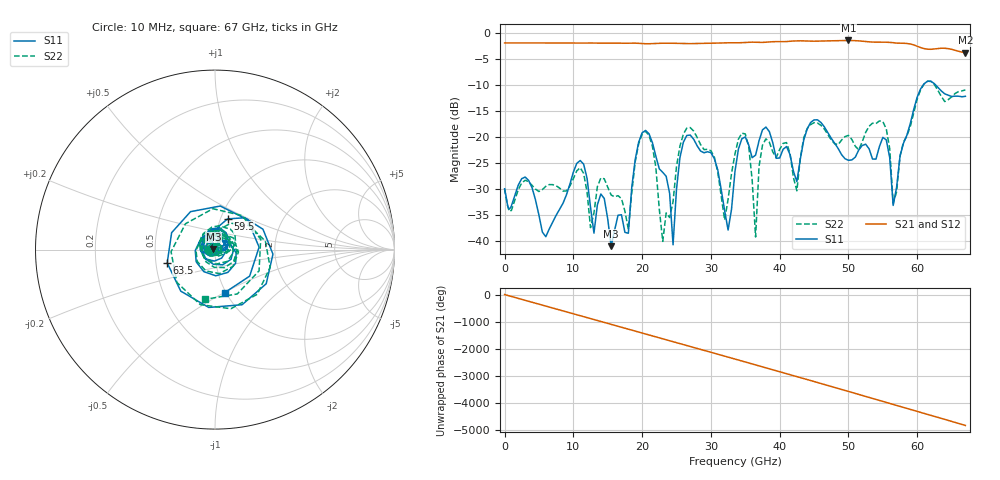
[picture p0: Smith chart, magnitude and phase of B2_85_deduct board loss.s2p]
!Keysight Technologies,N5247B,MY61255065,A.16.20.04
!Date: Sunday, September 03, 2023 22:00:42
!Correction: S11(C  2-Port  )
!S21(C  2-Port  )
!S12(C  2-Port  )
!S22(C  2-Port  )
!S2P File: Measurements: S11, S21, S12, S22:
!Deduct Board Loss
# Hz S  dB  R 50
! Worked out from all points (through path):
!   142 points, 10 MHz to 67 GHz, reference 50 ohm
!   highest |S21| = -1.48 dB at 50 GHz (marker M1); lowest = -3.8 dB at 67 GHz (marker M2)
!   lowest |S11| = -41.0 dB at 15.5 GHz (marker M3), VSWR 1.02, Z = 49.2 + j0.298 ohm
!   |S11| at or under -10 dB: start of sweep to 60.89 GHz; 62.66 GHz to end of sweep
!   |S22| runs from -40.0 to -9.3 dB; largest |S21 - S12| = 0.0028
!   S11 on the Smith chart (normalised r, x): 10 MHz: 0.94, -0.00; 59.5 GHz: 1.08, +0.38; 63.5 GHz: 0.57, -0.09; 67 GHz: 0.99, -0.50
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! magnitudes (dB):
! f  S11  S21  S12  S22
! 10 MHz  -29.9  -2.0  -1.9  -29.9
! 6 GHz  -39.1  -2.0  -2.0  -29.5
! 11.5 GHz  -25.2  -2.0  -2.0  -27.0
! 15.5 GHz  -41.0  -2.0  -2.0  -31.1
! 18 GHz  -38.5  -2.0  -2.0  -37.7
! 20.5 GHz  -18.7  -2.1  -2.1  -18.9
! 22.5 GHz  -26.1  -2.0  -2.0  -33.9
! 24.5 GHz  -40.7  -2.0  -2.0  -32.4
! 26.5 GHz  -19.7  -2.1  -2.1  -18.3
! 32 GHz  -34.2  -1.9  -1.9  -35.9
! 34 GHz  -22.3  -1.9  -1.9  -20.4
! 35.5 GHz  -21.5  -1.8  -1.8  -21.9
! 36.5 GHz  -23.5  -1.8  -1.8  -39.2
! 37.5 GHz  -18.6  -1.9  -1.8  -21.6
! 42.5 GHz  -28.6  -1.6  -1.6  -30.3
! 45 GHz  -16.7  -1.6  -1.6  -17.3
! 50 GHz  -24.5  -1.5  -1.5  -19.7
! 56 GHz  -24.0  -1.8  -1.8  -22.3
! 56.5 GHz  -33.1  -1.9  -1.9  -32.7
! 59.5 GHz  -14.6  -2.3  -2.3  -15.3
! 63.5 GHz  -11.2  -3.0  -2.9  -12.2
! 67 GHz  -12.2  -3.8  -3.8  -11.0
